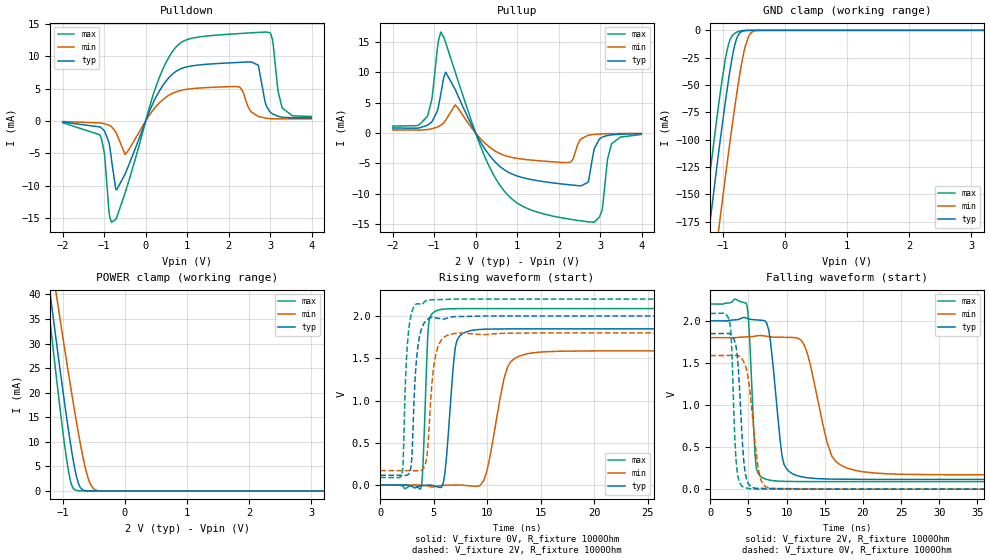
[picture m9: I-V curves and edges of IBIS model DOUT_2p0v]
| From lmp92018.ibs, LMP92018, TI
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|   Model
[Model]   DOUT_2p0v
Model_type   3-state
Polarity   Non-Inverting
Vmeas = 1
Vref = 0
Cref = 1pF
Rref = 1000000
|   typ   min   max
C_comp   0.5310pF   0.5030pF   0.6389pF
[Voltage Range]   2   1.8   2.2
[Temperature Range]   27   125   -40
[Pullup Reference]   2   1.8   2.2
[Pulldown Reference]   0   0   0
[Power Clamp Reference]   2   1.8   2.2
[GND Clamp Reference]   0   0   0
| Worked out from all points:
|   slope of the pulldown table from 0 to 0.3 V, typ, clamps not added: 69.9 ohm
|   slope of the pullup table from 0 to 0.3 V, typ, clamps not added: 89.5 ohm
|   GND clamp passes 1 mA (typ) near -0.69 V on its own axis
|   POWER clamp passes 1 mA (typ) near -0.73 V on its own axis
|   falling waveform, V_fixture 2V, R_fixture 1000Ohm: 20-80 % time 1.23ns typ, 2.41ns min, 650ps max; typ from 2 V to 0.116 V
|   rising waveform, V_fixture 0V, R_fixture 1000Ohm: 20-80 % time 662ps typ, 1.37ns min, 359ps max; typ from 0 V to 1.85 V
|   rising waveform, V_fixture 2V, R_fixture 1000Ohm: 20-80 % time 492ps typ, 618ps min, 417ps max; typ from 0.116 V to 2 V
|   falling waveform, V_fixture 0V, R_fixture 1000Ohm: 20-80 % time 720ps typ, 1.13ns min, 513ps max; typ from 1.85 V to 0 V
[Pulldown]
|   Voltage   I(typ)   I(min)   I(max)
-2V       -164.6uA   -79.4uA    -265.5uA
-1.106V   -915.6uA   -304.7uA   -2.129mA
-818mV    -6.269mA   -904.2uA   -15.65mA
-698mV    -10.65mA   -2.025mA   -14.91mA
-494mV    -8.178mA   -5.202mA   -11.08mA
346mV     4.811mA    2.898mA    6.983mA
934mV     8.273mA    4.842mA    12.42mA
2.254V    9.059mA    5.256mA    13.52mA
2.71V     8.65mA     721.9uA    13.69mA
2.986V    1.507mA    379uA      13.66mA
3.286V    580.8uA    338.6uA    2.146mA
3.994V    512.3uA    339uA      693.8uA
[GND Clamp]
|   Voltage   I(typ)   I(min)   I(max)
-2V       -557.2mA   -628.1mA   -512.8mA
-1.562V   -344.7mA   -416.3mA   -299.5mA
-1.262V   -202mA     -273.8mA   -156.6mA
-1.25V    -196.3mA   -268.2mA   -151mA
-1.046V   -103.3mA   -173.9mA   -59.81mA
-962mV    -67.33mA   -136.3mA   -27.86mA
-902mV    -43.61mA   -110.1mA   -11.85mA
-782mV    -8.626mA   -60.87mA   -1.933mA
-638mV    -299.9uA   -14.77mA   -73.21uA
-566mV    -48.54uA   -3.762mA   -7.764uA
-482mV    -4.863uA   -446.4uA   0A
3.994V    0A         0A         0A
[Pullup]
|   Voltage   I(typ)   I(min)   I(max)
-2V       841.5uA    530.7uA    1.162mA
-1.166V   1.299mA    581.9uA    2.744mA
-842mV    6.387mA    1.288mA    16.66mA
-722mV    10.05mA    2.14mA     14.88mA
-494mV    7.206mA    4.654mA    10.09mA
322mV     -3.56mA    -2.239mA   -5.416mA
1.186V    -7.425mA   -4.337mA   -12.24mA
2.542V    -8.698mA   -947uA     -14.47mA
2.866V    -2.463mA   -206.6uA   -14.65mA
3.046V    -678.3uA   -132uA     -12.76mA
3.274V    -293.3uA   -87.56uA   -1.844mA
3.994V    -87.4uA    -39.48uA   -224.3uA
[POWER Clamp]
|   Voltage   I(typ)   I(min)   I(max)
-2V       120.2mA    116.5mA    127.3mA
-1.286V   48.53mA    55.58mA    44.02mA
-1.19V    38.98mA    47.39mA    33mA
-1.106V   30.76mA    40.29mA    23.59mA
-914mV    12.93mA    24.49mA    4.521mA
-866mV    8.929mA    20.69mA    1.596mA
-806mV    4.555mA    16.07mA    247uA
-722mV    809.1uA    10.01mA    24.36uA
-614mV    25.92uA    3.608mA    0A
-530mV    0A         842.3uA    0A
-458mV    0A         147.1uA    0A
3.994V    0A         0A         0A
[Ramp]
R_load = 1000
|   typ   min   max
dV/dt_r   1.10854/6.62133e-10   0.952238/1.3727e-09   1.25228/3.58625e-10
dV/dt_f   1.13052/1.22712e-09   0.977469/2.40907e-09   1.26637/6.49525e-10
[Falling Waveform]
V_fixture = 2V
V_fixture_min = 1.8V
V_fixture_max = 2.2V
R_fixture = 1000Ohm
C_fixture = 0F
|   Time   V(typ)   V(min)   V(max)
0s        2V         1.8V       2.2V
4.793ns   2.031V     1.809V     2.186V
5.048ns   2.024V     1.81V      1.963V
6.041ns   2.011V     1.821V     246.8mV
7.62ns    1.903V     1.814V     110mV
9.402ns   395.4mV    1.805V     93.84mV
12.01ns   145.5mV    1.755V     90.31mV
15.95ns   119.7mV    387.9mV    89.5mV
18.89ns   117.3mV    224.6mV    89.5mV
100ns     115.8mV    170.9mV    89.39mV
[Rising Waveform]
V_fixture = 0V
V_fixture_min = 0V
V_fixture_max = 0V
R_fixture = 1000Ohm
C_fixture = 0F
|   Time   V(typ)   V(min)   V(max)
0s        135nV      83.69nV    -457.5nV
3.804ns   -8.093mV   -2.068mV   -39.55mV
4.517ns   40.44uV    -13.22mV   1.903V
5.699ns   -25.47mV   -6.271mV   2.077V
7.032ns   1.638V     -350.5uV   2.086V
8.602ns   1.831V     -12.55mV   2.087V
9.995ns   1.844V     176.8mV    2.087V
11.91ns   1.847V     1.397V     2.087V
14.21ns   1.847V     1.562V     2.087V
100ns     1.848V     1.587V     2.087V
[Rising Waveform]
V_fixture = 2V
V_fixture_min = 1.8V
V_fixture_max = 2.2V
R_fixture = 1000Ohm
C_fixture = 0F
|   Time   V(typ)   V(min)   V(max)
0s        115.8mV    170.9mV    89.39mV
2.028ns   114.8mV    169.8mV    130.6mV
2.134ns   114.7mV    169.8mV    250.7mV
2.45ns    114.6mV    169.6mV    1.49V
2.814ns   176.3mV    169.4mV    1.97V
3.492ns   1.611V     169mV      2.145V
4.431ns   1.962V     433.3mV    2.188V
5.17ns    1.978V     1.529V     2.192V
6.944ns   1.992V     1.792V     2.199V
100ns     2V         1.8V       2.2V
[Falling Waveform]
|Gnd
V_fixture = 0V
V_fixture_min = 0V
V_fixture_max = 0V
R_fixture = 1000Ohm
C_fixture = 0F
|   Time   V(typ)   V(min)   V(max)
0s        1.848V     1.587V     2.087V
2.549ns   1.846V     1.589V     1.978V
2.764ns   1.827V     1.589V     1.767V
3.199ns   1.757V     1.589V     638.8mV
3.424ns   1.667V     1.589V     299.4mV
4.517ns   235.2mV    1.486V     17.72mV
5.17ns    43.76mV    1.185V     6.525mV
6.421ns   9.925mV    183mV      1.65mV
7.936ns   7.32mV     9.542mV    533.5uV
100ns     137.6nV    85.18nV    -466.7nV
